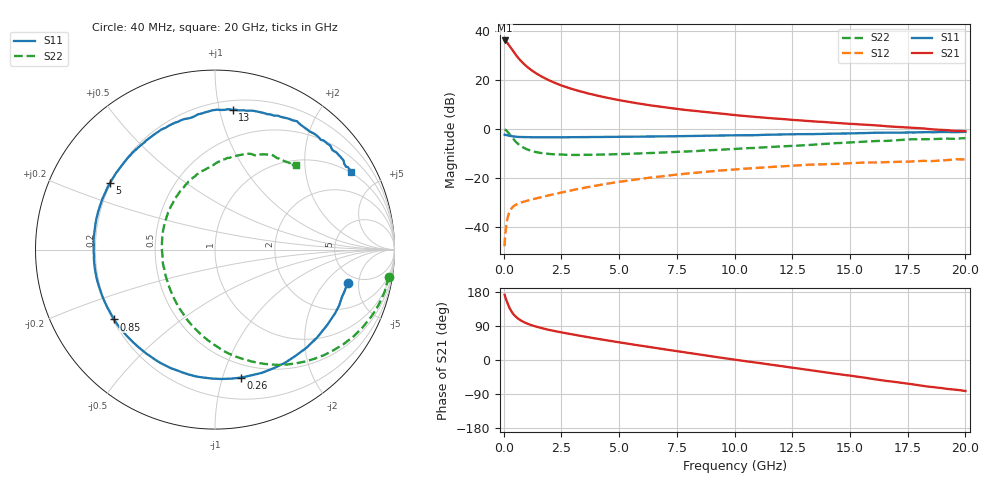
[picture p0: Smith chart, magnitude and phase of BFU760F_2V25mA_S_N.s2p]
! Filename:  P:\Prog\Test\Noise\ATS_data\Testdata_Net\BFU760\BFU760F_2W_C1_2V25mA_D.s2p
! Date/Time: Mon 06/Feb/2012 15:05:42
! BFU760_2W_C1_2V25mA
! bias mode 1: Vout= 2.0002 V, Iout=24.9750 mA, Vin= 0.7911 V, Iin= 0.0805 mA
! Date/time Fri Mar 18 14:53:56 2011
! Device data file deembeded for feedlines and parallel
! Original file: \BFU760\BFU760_2W_C1_2V25mA_R.s2p
! Feed-files: PR003V01_101208_Feed1.s2p, PR003V01_101208_Feed2.s2p
! Parallel-file: PR003V01_101208_Par.s2p
# MHz S MA R 50
!  Freq-MHz  S11-mag  S11-arg  S21-mag  S21-arg  S12-mag  S12-arg  S22-mag  S22-arg
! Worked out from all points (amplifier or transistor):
!   167 points, 40 MHz to 20 GHz, reference 50 ohm
!   highest |S21| = 36.3 dB at 40 MHz (marker M1)
!   |S21| within 3 dB of that: start of sweep to 310.6 MHz
!   unconditionally stable (mu >= 1): 4.004 GHz to 13.87 GHz
!   at 550 MHz: K = 0.29, MSG = 30.5 dB, |S12| = -30.9 dB
!   at 4.2 GHz: K = 1.01, MAG = 17.5 dB, |S12| = -22.9 dB
!   at 20 GHz: K = 0.91, MSG = 5.8 dB, |S12| = -12.4 dB
!   lowest NFmin = 0.55 dB at 400 MHz
!   S11 on the Smith chart (normalised r, x): 40 MHz: 4.11, -3.63; 260 MHz: 0.38, -1.15; 850 MHz: 0.21, -0.30; 5 GHz: 0.20, +0.28; 13 GHz: 0.27, +1.10; 20 GHz: 0.96, +3.53
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40  0.7626 -14.0  65.24 172.2  0.003986 81.9  0.9799 -8.9
50  0.7575 -18.4  64.94 169.6  0.005378 83.6  0.9754 -11.6
90  0.7538 -31.2  63.07 162.3  0.008801 75.4  0.9549 -21.0
140  0.7475 -46.9  59.73 153.7  0.01299 68.6  0.9105 -32.2
200  0.737 -64.0  54.87 144.5  0.01721 61.5  0.8449 -44.1
260  0.7279 -78.7  50.08 136.6  0.02048 55.7  0.777 -54.7
300  0.7218 -87.2  46.89 132.1  0.02219 52.4  0.7347 -61.0
380  0.711 -102.0  41.39 124.3  0.02489 47.5  0.6556 -71.9
500  0.6984 -118.2  34.36 115.7  0.02764 42.5  0.5652 -85.3
650  0.6886 -132.3  27.94 108.0  0.02997 39.2  0.4846 -98.4
850  0.6841 -145.3  22.14 100.7  0.03225 37.4  0.4181 -112.1
1250  0.6788 -161.1  15.47 91.1  0.03637 37.4  0.3512 -131.5
1800  0.677 -174.1  10.86 81.8  0.04211 39.2  0.3146 -149.4
2450  0.6779 175.8  7.973 73.4  0.04945 40.8  0.3005 -163.9
3400  0.6828 164.1  5.769 62.9  0.06144 40.8  0.2959 -179.0
5000  0.6926 147.7  3.909 46.6  0.08288 37.0  0.3062 161.3
6800  0.7063 131.9  2.86 29.8  0.1071 29.4  0.3289 143.7
10200  0.7458 104.4  1.893 -0.7  0.1509 10.4  0.3965 114.5
13000  0.7844 82.7  1.481 -24.5  0.183 -7.3  0.4657 92.9
13400  0.7866 80.2  1.437 -27.8  0.1869 -10.4  0.4778 90.0
16800  0.8434 54.3  1.12 -56.7  0.2111 -32.2  0.5784 65.2
20000  0.8744 29.7  0.9052 -81.8  0.2388 -53.8  0.6509 46.3
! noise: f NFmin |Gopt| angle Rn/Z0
400  0.5459  0.175  165.2  0.04197
700  0.5472  0.191  165.5  0.04309
1100  0.5516  0.2117  166.7  0.04437
1500  0.5591  0.2319  168.5  0.04543
1900  0.5698  0.2517  170.9  0.04625
2350  0.5855  0.2742  174.1  0.0469
3000  0.6151  0.3081  179.3  0.04733
3800  0.663  0.3542  186.5  0.047
4600  0.7232  0.4084  193.9  0.04576
6000  0.8588  0.5306  206.3  0.04134
